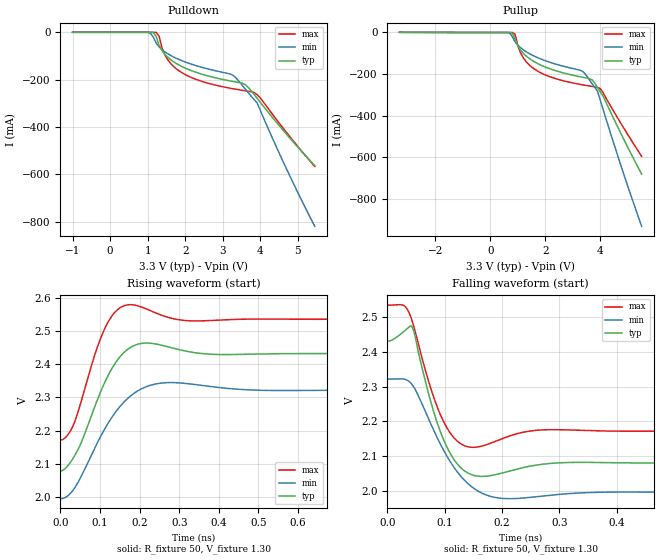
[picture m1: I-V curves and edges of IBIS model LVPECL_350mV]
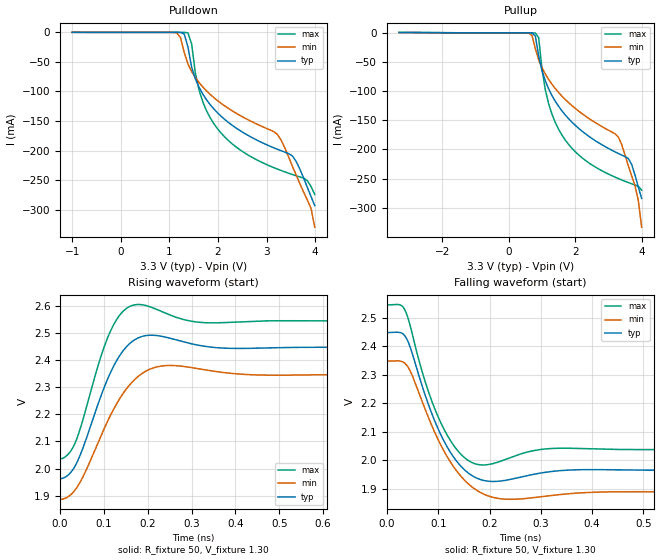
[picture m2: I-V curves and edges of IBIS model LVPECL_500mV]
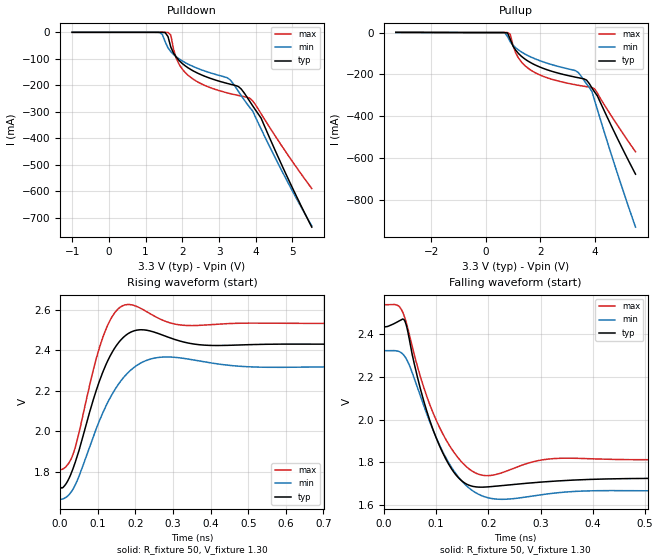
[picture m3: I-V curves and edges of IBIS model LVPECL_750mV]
|   This file is an IBIS representation of the   |
|   Integrated Device Technology Inc   |
|   8V49NS0312   |
|   FEMTOCLOCK NG CLOCK GENERATOR WITH 4 DIVIDERS   |
[IBIS Ver]   4.1
[File name]   8v49ns0312.ibs
[File Rev]   1.1
|Rev 1.1
|  Updated SDATA pin to I/O
|  Updated SCL Pin to SERIAL_IN
|Rev 1.0 Original, 13 Jun 2016
[Date]   01 Nov 2017
[Source]   Originated at Integrated Device Technology, Inc.
[Disclaimer]
IDT hereby grants the user of this IBIS model a non-exclusive,
nontransferable license to use this IBIS model under the following terms.
Before using this IBIS model, the user should read this license.
If the user does not accept these terms,  the IBIS model should be
returned to IDT within 30 days.
   The user is granted this license only to use the IBIS model and
is not granted rights to sell, load, rent, lease or license the IBIS
model in whole or in part, or in modified form to anyone other than
user. User may modify the IBIS model to suit its specific
applications but rights to derivative works and such modifications
shall belong to IDT.
   This IBIS model is provided on an "AS IS" basis and IDT makes
absolutely no warranty with respect to the information contained
herein. IDT DISCLAIMS AND CUSTOMER WAIVES ALL WARRANTIES, EXPRESS
OR IMPLIED, INCLUDING WARRANTIES OF MERCHANTABILITY OR FITNESS FOR
A PARTICULAR PURPOSE. The entire risk as to quality and performance
is with the Customer. ACCORDINGLY, IN NO EVENT SHALL THE COMPANY BE
LIABLE FOR ANY DAMAGES, WHETHER IN CONTRACT OR TORT,INCLUDING ANY
LOST PROFITS OR OTHER INCIDENTAL, CONSEQUENTIAL, EXEMPLARY, OR
PUNITIVE DAMAGES ARISING OUT OF THE USE OR APPLICATION OF THE IBIS
model provided in this package. Further, IDT reserves the right to
make changes without notice to any product herein to improve
reliability, function, or design. IDT does not convey any license
under patent rights or any other intellectual property rights,
including those of third parties.
   IDT is not obligated to provide maintenance or support
for the licensed IBIS model.
[Copyright] Copyright 2015 by Integrated Device Technology, Inc.
[Component]   8V49NS0312NLGI
[Manufacturer] Integrated Device Technology, Inc.
[Package]
|LD QFN 64
|lead + wire
|   Typ   Min   Max
R_pkg   0.15994   0.09324   0.20004
L_pkg   2.530359n   1.8988n   3.1063n
C_pkg   0.078001p   0.067589p   0.11523p
[Pin] signal_name model_name   R_pin   L_pin   C_pin
1  VCCOB   POWER   1.6449E-01   2.956n   0.08458p
2  QB0   LVDS_LVPECL_0312   1.9750E-01   2.7461n   0.088784p
3  nQB0   LVDS_LVPECL_0312   1.7981E-01   2.699n   0.082304p
4  QB1   LVDS_LVPECL_0312   1.7541E-01   2.4836n   0.082529p
5  nQB1   LVDS_LVPECL_0312   1.5766E-01   2.437n   0.075279p
6  QB2   LVDS_LVPECL_0312   1.4595E-01   2.3494n   0.071373p
7  nQB2   LVDS_LVPECL_0312   1.4009E-01   2.2382n   0.070004p
8  QB3   LVDS_LVPECL_0312   1.4152E-01   2.1201n   0.069711p
9  nQB3   LVDS_LVPECL_0312   1.4111E-01   2.1159n   0.069506p
10 VCCOB   POWER   1.3903E-01   2.2556n   0.069921p
11 ND[0]   RF_INESD_200_PUP   1.4414E-01   2.3769n   0.069368p
12 NC[1]   RF_INESD_200_PUP   1.4772E-01   2.3318n   0.070114p
13 VCCOD   POWER   1.5989E-01   2.3679n   0.077159p
14 QD1   RF_COUT_9F_7F_SE   1.6857E-01   2.5122n   0.077263p
15 QD0   LVDS_LVPECL_0312   1.6231E-01   2.543n   0.081562p
16 nQD0   LVDS_LVPECL_0312   1.3552E-01   2.8375n   0.077893p
17 NB[0]   RF_INESD_200_PUP   1.3290E-01   2.7501n   0.074621p
18 NB[1]   RF_INESD_200_PUP   1.8095E-01   2.7617n   0.08237p
19 NC[0]   RF_INESD_200_PUP   1.6926E-01   2.5289n   0.080624p
20 NC[1]   RF_INESD_200_PUP   1.6506E-01   2.3465n   0.075995p
21 VCCA_IN1   POWER   1.5450E-01   2.3031n   0.072045p
22 NA[1]   RF_INESD_200_PUP   1.4838E-01   2.1982n   0.072043p
23 CAPBIAS   NC   1.3877E-01   2.2149n   0.068646p
24 VCCA_IN2   POWER   1.3433E-01   2.1808n   0.068017p
25 CR   NC   1.4411E-01   2.1294n   0.070068p
26 CAPREG   NC   1.4387E-01   2.2043n   0.071183p
27 LFFR   NC   1.5194E-01   2.3838n   0.071178p
28 LFF   NC   1.5971E-01   2.3509n   0.075039p
29 VCCA   POWER   1.7026E-01   2.5352n   0.080161p
30 NC   NC   1.8017E-01   2.758n   0.086153p
31 VCC_CP   POWER   9.3242E-02   1.8988n   0.11523p
32 ICP   NC   1.3198E-01   2.7827n   0.071584p
33 VCCOC   POWER   1.6203E-01   3.0318n   0.081581p
34 nQC1   LVDS_LVPECL_0312   1.9612E-01   2.7713n   0.087674p
35 QC1   LVDS_LVPECL_0312   1.8463E-01   2.711n   0.082141p
36 nQC0   LVDS_LVPECL_0312   1.7410E-01   2.5236n   0.081436p
37 QC0   LVDS_LVPECL_0312   1.5857E-01   2.4566n   0.075124p
38 VCCOC   POWER   1.4575E-01   2.3561n   0.072098p
39 VCCOA   POWER   1.4055E-01   2.251n   0.070146p
40 nQA3   LVDS_LVPECL_0312   1.4352E-01   2.1244n   0.068826p
41 QA3   LVDS_LVPECL_0312   1.4468E-01   2.1039n   0.069621p
42 nQA2   LVDS_LVPECL_0312   1.3923E-01   2.2333n   0.067589p
43 QA2   LVDS_LVPECL_0312   1.4807E-01   2.2049n   0.069987p
44 nQA1   LVDS_LVPECL_0312   1.5598E-01   2.3003n   0.074857p
45 QA1   LVDS_LVPECL_0312   1.6074E-01   2.5324n   0.077114p
46 nQA0   LVDS_LVPECL_0312   1.7421E-01   2.6897n   0.082311p
47 QA0   LVDS_LVPECL_0312   2.0004E-01   2.7944n   0.09063p
48 VCCOA   POWER   1.6631E-01   3.0273n   0.085515p
49 REF_SEL   RF_INESD_200_PD   1.5017E-01   3.0793n   0.080972p
50 VCC_CK   POWER   1.7648E-01   2.7832n   0.08889p
51 nCLK   RF_INESD_200_PUP   1.9178E-01   2.7299n   0.087693p
52 CLK   RF_INESD_200_PD   1.7825E-01   2.7642n   0.082129p
53 FIN[1]   RF_INESD_200_PUP   1.6637E-01   2.7168n   0.080022p
54 FIN[0]   RF_INESD_200_PUP   1.6226E-01   2.6712n   0.0769p
55 CAPXTAL   NC   1.5685E-01   2.6157n   0.07263p
56 OSCO   NC   1.6928E-01   2.4353n   0.077211p
57 OSCI   NC   1.6908E-01   2.4716n   0.079042p
58 VCCA_XT   POWER   1.6376E-01   2.5979n   0.078197p
59 NA[0]   RF_INESD_200_PUP   1.7407E-01   2.5694n   0.081073p
60 RES   NC   1.7923E-01   2.6937n   0.079745p
61 SDATA   SERIAL_IO   1.7655E-01   2.8937n   0.079001p
62 SCLK   SERIAL_IN   1.8689E-01   2.9915n   0.086026p
63 VCC_SP   POWER   1.7813E-01   3.1063n   0.089577p
64 LOCK   RF_COUT_12F_IO   1.6199E-01   3.0138n   0.083996p
[Diff Pin]   inv_pin vdiff   tdelay_typ   tdelay_min   tdelay_max
| Inputs
52   51   0.2   NA   NA   NA
|Outputs
2   3   NA   0   0   0
4   5   NA   0   0   0
6   7   NA   0   0   0
8   9   NA   0   0   0
15   16   NA   0   0   0
47   46   NA   0   0   0
45   44   NA   0   0   0
43   42   NA   0   0   0
41   40   NA   0   0   0
37   36   NA   0   0   0
35   34   NA   0   0   0
[Model Selector] LVDS_LVPECL_0312
LVDS_350mV   350mV LVDS Model
LVDS_500mV   500mV LVDS Model
LVDS_750mV   750mV LVDS Model
LVPECL_350mV   350mV LVPECL Model
LVPECL_500mV   500mV LVPECL Model
LVPECL_750mV   750mV LVPECL Model
| Models and submodels in the file (12): LVPECL_350mV (Output_ECL), LVPECL_500mV (Output_ECL), LVPECL_750mV (Output_ECL), LVDS_350mV (Output), LVDS_500mV (Output), LVDS_750mV (Output), RF_INESD_200_PUP (Input), RF_COUT_9F_7F_SE (Output), RF_INESD_200_PD (Input), RF_COUT_12F_IO (Output), SERIAL_IO (I/O_open_drain), SERIAL_IN (Input)
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[Model]   LVPECL_350mV
Model_type   Output_ECL
Polarity   Non-Inverting
|   typ   min   max
C_comp   2pF   1.5pF   2.5pF
Vmeas= 2.244V
Rref = 50
Cref = 0
Vref = 1.3V
|   typ   min   max
[Voltage range]   3.3V   3.135V   3.465V
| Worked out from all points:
|   rising waveform, R_fixture 50, V_fixture 1.30: 20-80 % time 71.2ps typ, 87.9ps min, 55.4ps max; typ from 2.08 V to 2.43 V
|   falling waveform, R_fixture 50, V_fixture 1.30: 20-80 % time 37.7ps typ, 60.2ps min, 38.3ps max; typ from 2.43 V to 2.08 V
[Pulldown]
|Voltage   I (typ)   I (min)   I (max)
-1V       46.99uA    55.49uA    39.05uA
996mV     -2.417uA   -292.3uA   -6.854nA
1.226V    -17.75mA   -46.05mA   -610.7uA
1.303V    -54.71mA   -61.43mA   -16.42mA
1.38V     -76.94mA   -72.91mA   -65.09mA
1.533V    -105.1mA   -90.45mA   -115.9mA
1.84V     -139mA     -115.4mA   -163.4mA
3.299V    -208.7mA   -185mA     -239.4mA
3.606V    -222.3mA   -241.7mA   -247.6mA
3.913V    -278.8mA   -298.2mA   -263.6mA
4.681V    -427.9mA   -572.1mA   -420.1mA
5.448V    -563mA     -819.9mA   -567.2mA
[Pullup]
|Voltage   I (typ)   I (min)   I (max)
-3.3V     781.4uA    613.4uA    1.002mA
600mV     -980.9nA   -86.79uA   -5.239nA
800mV     -2.307mA   -19.53mA   -84.09uA
900mV     -32.62mA   -44.9mA    -8.184mA
1V        -64.66mA   -60.7mA    -61.81mA
1.2V      -100.1mA   -83.16mA   -121.4mA
1.6V      -140.4mA   -113.6mA   -175.2mA
3.4V      -216.2mA   -191.5mA   -252.3mA
3.7V      -227.4mA   -246mA     -258.9mA
3.9V      -265.1mA   -282.8mA   -263.2mA
4.1V      -304.9mA   -369.6mA   -289.4mA
5.5V      -679.8mA   -930.4mA   -594.4mA
[Ramp]
|   typ   min   max
dV/dt_r   0.23/0.08n   0.209/0.098n   0.244/0.064n
dV/dt_f   0.26/0.047n   0.207/0.066n   0.247/0.046n
R_load =   50.0000
[Rising Waveform]
R_fixture = 50
V_fixture = 1.30   | VCC_typ - 2V
V_fixture_max = 1.465   | VCC_max - 2V
V_fixture_min = 1.135   | VCC_min - 2V
C_fixture = 0.0p
| Time   typ   min   max
0s        2.08V      1.995V     2.172V
34.03ps   2.121V     2.024V     2.221V
88.09ps   2.277V     2.151V     2.433V
114.1ps   2.351V     2.21V      2.512V
140.1ps   2.406V     2.257V     2.559V
168.2ps   2.443V     2.295V     2.578V
212.2ps   2.463V     2.33V      2.568V
276.3ps   2.451V     2.344V     2.539V
406.4ps   2.429V     2.329V     2.533V
2ns       2.431V     2.322V     2.535V
[Falling Waveform]
R_fixture = 50
V_fixture = 1.30   | VCC_typ - 2V
V_fixture_max = 1.465   | VCC_max - 2V
V_fixture_min = 1.135   | VCC_min - 2V
C_fixture = 0.0p
| Time   typ   min   max
0s        2.432V     2.322V     2.535V
30.03ps   2.461V     2.322V     2.533V
44.04ps   2.47V      2.304V     2.486V
72.07ps   2.279V     2.207V     2.315V
94.09ps   2.163V     2.129V     2.214V
118.1ps   2.086V     2.063V     2.149V
144.1ps   2.048V     2.015V     2.126V
194.2ps   2.049V     1.979V     2.146V
280.3ps   2.078V     1.986V     2.176V
2ns       2.08V      1.996V     2.172V
[Model]   LVPECL_500mV
Model_type   Output_ECL
Polarity   Non-Inverting
|   typ   min   max
C_comp   2pF   1.5pF   2.5pF
Vmeas= 2.203V
Rref = 50
Cref = 0
Vref = 1.3V
|   typ   min   max
[Voltage range]   3.3V   3.135V   3.465V
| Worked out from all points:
|   rising waveform, R_fixture 50, V_fixture 1.30: 20-80 % time 65.5ps typ, 80ps min, 55.1ps max; typ from 1.96 V to 2.45 V
|   falling waveform, R_fixture 50, V_fixture 1.30: 20-80 % time 59.8ps typ, 70.6ps min, 53.8ps max; typ from 2.45 V to 1.96 V
[Pulldown]
|Voltage   I (typ)   I (min)   I (max)
|Note, modeling breaks down at 250mA and above.  This is well beyond the functional   |
|operating range of the device.  Should this scenario occur, catastrophic failure and   |
|possible damage to the device and/or board is of higher concern than the I-V curve   |
|behavior.  The IBIS checker will flag currents in excess of 10A with warnings.  Lines   |
|with currents in excess of 0.35 A have been commented out.  The points still remain|
|available to the user if the user desires to use them.   |
|Note, modeling breaks down at 250mA and above.  This is well beyond the functional   |
|operating range of the device.  Should this scenario occur, catastrophic failure and   |
|possible damage to the device and/or board is of higher concern than the I-V curve   |
|behavior.  The IBIS checker will flag currents in excess of 10A with warnings.  Lines   |
|with currents in excess of 0.35 A have been commented out.  The points still remain|
|available to the user if the user desires to use them.   |
-1V       49.32uA    57.22uA    39.05uA
1.149V    -6.032uA   -1.009mA   -8.922nA
1.303V    -2.562mA   -33.63mA   -17.79uA
1.38V     -24.61mA   -53.43mA   -796.1uA
1.457V    -59.03mA   -66.37mA   -19.68mA
1.533V    -78.83mA   -76.55mA   -69.1mA
1.687V    -104.7mA   -92.49mA   -117.8mA
2.071V    -142.6mA   -120.6mA   -171.2mA
3.222V    -198mA     -172.8mA   -231.5mA
3.606V    -218.3mA   -241.5mA   -242.7mA
3.913V    -277.9mA   -297.8mA   -260.9mA
3.99V     -293.3mA   -329.8mA   -274.5mA
|| 4.06667e+00   -3.08432e-01   -3.67426e-01   -2.90478e-01
|| 4.14343e+00   -3.23924e-01   -4.05071e-01   -3.07173e-01
|| 4.22020e+00   -3.53714e-01   -4.42647e-01   -3.23828e-01
|| 4.29697e+00   -3.97748e-01   -4.80134e-01   -3.40232e-01
|| 4.37374e+00   -4.42041e-01   -5.17517e-01   -3.56685e-01
|| 4.45051e+00   -4.86426e-01   -5.54778e-01   -3.88442e-01
|| 4.52727e+00   -5.30804e-01   -5.91886e-01   -4.43339e-01
|| 4.60404e+00   -5.75132e-01   -5.91886e-01   -4.97475e-01
|| 4.68081e+00   -6.19384e-01   -5.91886e-01   -5.50215e-01
|| 4.75758e+00   -6.63538e-01   -5.91886e-01   -6.03199e-01
|| 4.83434e+00   -7.07558e-01   -5.91886e-01   -6.56255e-01
|| 4.91111e+00   -7.51390e-01   -5.91886e-01   -7.09286e-01
|| 4.98788e+00   -7.94950e-01   -5.91886e-01   -7.62250e-01
|| 5.06465e+00   -8.38293e-01   -5.91886e-01   -8.15110e-01
|| 5.14141e+00   -8.38293e-01   -5.91886e-01   -8.67827e-01
|| 5.21818e+00   -8.38293e-01   -5.91886e-01   -9.20344e-01
|| 5.29495e+00   -8.38293e-01   -5.91886e-01   -9.72672e-01
|| 5.37172e+00   -8.38293e-01   -5.91886e-01   -1.02500e+00
|| 5.44848e+00   -8.38293e-01   -5.91886e-01   -1.07696e+00
[Pullup]
|Voltage   I (typ)   I (min)   I (max)
|Note, modeling breaks down at 250mA and above.  This is well beyond the functional   |
|operating range of the device.  Should this scenario occur, catastrophic failure and   |
|possible damage to the device and/or board is of higher concern than the I-V curve   |
|behavior.  The IBIS checker will flag currents in excess of 10A with warnings.  Lines   |
|with currents in excess of 0.35 A have been commented out.  The points still remain|
|available to the user if the user desires to use them.   |
-3.3V     746.6uA    586.4uA    1.002mA
700mV     -165.7uA   -4.504mA   -647nA
800mV     -5.314mA   -26.92mA   -83.98uA
900mV     -39.18mA   -46.19mA   -8.176mA
1V        -64.77mA   -59.66mA   -61.8mA
1.2V      -95.95mA   -79.87mA   -121.4mA
1.7V      -140.7mA   -114.2mA   -183.7mA
3.3V      -206.9mA   -178.8mA   -249.9mA
3.6V      -215.6mA   -228mA     -256.8mA
3.8V      -243.9mA   -262.2mA   -261mA
3.9V      -264.5mA   -287.2mA   -263.2mA
4V        -283.9mA   -333.3mA   -269.8mA
| 4.10000e+00   -3.02415e-01   -3.78849e-01   -2.89415e-01
| 4.20000e+00   -3.40057e-01   -4.23937e-01   -3.13568e-01
| 4.30000e+00   -3.94775e-01   -4.68570e-01   -3.35833e-01
| 4.40000e+00   -4.49108e-01   -4.68570e-01   -3.56546e-01
| 4.50000e+00   -5.03021e-01   -4.68570e-01   -4.17084e-01
| 4.60000e+00   -5.56418e-01   -4.68570e-01   -4.85623e-01
| 4.70000e+00   -6.09244e-01   -4.68570e-01   -5.54012e-01
| 4.80000e+00   -6.61642e-01   -4.68570e-01   -6.22199e-01
| 4.90000e+00   -7.13735e-01   -4.68570e-01   -6.90136e-01
| 5.00000e+00   -7.13735e-01   -4.68570e-01   -7.57722e-01
| 5.10000e+00   -7.13735e-01   -4.68570e-01   -8.24630e-01
| 5.20000e+00   -7.13735e-01   -4.68570e-01   -8.90368e-01
| 5.30000e+00   -7.13735e-01   -4.68570e-01   -9.55440e-01
| 5.40000e+00   -7.13735e-01   -4.68570e-01   -1.02066e+00
| 5.50000e+00   -7.13735e-01   -4.68570e-01   -1.08596e+00
[Ramp]
|   typ   min   max
dV/dt_r   0.316/0.074n   0.295/0.088n   0.34/0.064n
dV/dt_f   0.314/0.068n   0.291/0.077n   0.338/0.064n
R_load =   50.0000
[Rising Waveform]
R_fixture = 50
V_fixture = 1.30   | VCC_typ - 2V
V_fixture_max = 1.465   | VCC_max - 2V
V_fixture_min = 1.135   | VCC_min - 2V
C_fixture = 0.0p
| Time   typ   min   max
0s        1.963V     1.887V     2.036V
20.02ps   1.979V     1.898V     2.056V
36.04ps   2.015V     1.925V     2.101V
92.09ps   2.263V     2.117V     2.408V
118.1ps   2.365V     2.207V     2.518V
142.1ps   2.431V     2.273V     2.577V
170.2ps   2.474V     2.328V     2.603V
234.2ps   2.486V     2.378V     2.577V
340.3ps   2.448V     2.361V     2.537V
2ns       2.446V     2.346V     2.544V
[Falling Waveform]
R_fixture = 50
V_fixture = 1.30   | VCC_typ - 2V
V_fixture_max = 1.465   | VCC_max - 2V
V_fixture_min = 1.135   | VCC_min - 2V
C_fixture = 0.0p
| Time   typ   min   max
0s        2.448V     2.348V     2.545V
26.03ps   2.448V     2.348V     2.545V
36.04ps   2.433V     2.338V     2.523V
80.08ps   2.199V     2.153V     2.244V
118.1ps   2.044V     2.01V      2.086V
148.1ps   1.971V     1.935V     2.013V
180.2ps   1.933V     1.888V     1.984V
234.2ps   1.93V      1.863V     2.005V
336.3ps   1.963V     1.879V     2.042V
2ns       1.964V     1.888V     2.037V
[Model]   LVPECL_750mV
Model_type   Output_ECL
Polarity   Non-Inverting
|   typ   min   max
C_comp   2pF   1.5pF   2.5pF
Vmeas= 2.084V
Rref = 50
Cref = 0
Vref = 1.3V
|   typ   min   max
[Voltage range]   3.3V   3.135V   3.465V
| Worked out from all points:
|   rising waveform, R_fixture 50, V_fixture 1.30: 20-80 % time 69.3ps typ, 86ps min, 55.4ps max; typ from 1.73 V to 2.43 V
|   falling waveform, R_fixture 50, V_fixture 1.30: 20-80 % time 52.9ps typ, 66ps min, 58.3ps max; typ from 2.43 V to 1.73 V
[Pulldown]
|Voltage   I (typ)   I (min)   I (max)
-1V       46.99uA    52.79uA    34.37uA
1.38V     -1.938uA   -734uA     -1.297nA
1.457V    -46.63uA   -8.101mA   -69.37nA
1.61V     -15.95mA   -58.81mA   -244.4uA
1.687V    -55.72mA   -73.05mA   -10.72mA
1.84V     -94.89mA   -92.95mA   -100.1mA
2.147V    -133.2mA   -119.4mA   -161mA
3.222V    -193mA     -171.6mA   -228.6mA
3.529V    -204.9mA   -223.5mA   -238.6mA
3.913V    -276.9mA   -296.7mA   -258.7mA
4.143V    -323.6mA   -364.6mA   -307mA
5.525V    -736mA     -731.5mA   -590.1mA
[Pullup]
|Voltage   I (typ)   I (min)   I (max)
-3.3V     781.4uA    613.4uA    1.002mA
600mV     -965.4nA   -83.72uA   -5.214nA
800mV     -2.274mA   -19.17mA   -83.69uA
900mV     -32.44mA   -44.7mA    -8.155mA
1V        -64.57mA   -60.56mA   -61.77mA
1.2V      -100mA     -83.07mA   -121.4mA
1.6V      -140.4mA   -113.6mA   -175.2mA
3.4V      -216.2mA   -191.4mA   -252.3mA
3.7V      -227.4mA   -245.4mA   -258.9mA
3.9V      -265.1mA   -282.1mA   -263.2mA
4.1V      -303.3mA   -369mA     -289.4mA
5.5V      -677.6mA   -930.8mA   -570.3mA
[Ramp]
|   typ   min   max
dV/dt_r   0.468/0.08n   0.421/0.097n   0.489/0.065n
dV/dt_f   0.47/0.059n   0.416/0.072n   0.478/0.07n
R_load =   50.0000
[Rising Waveform]
R_fixture = 50
V_fixture = 1.30   | VCC_typ - 2V
V_fixture_max = 1.465   | VCC_max - 2V
V_fixture_min = 1.135   | VCC_min - 2V
C_fixture = 0.0p
| Time   typ   min   max
0s        1.725V     1.665V     1.811V
36.04ps   1.826V     1.721V     1.897V
92.09ps   2.181V     1.995V     2.332V
120.1ps   2.323V     2.119V     2.497V
146.1ps   2.415V     2.209V     2.588V
174.2ps   2.474V     2.278V     2.625V
244.2ps   2.493V     2.359V     2.576V
340.3ps   2.436V     2.357V     2.523V
548.5ps   2.43V      2.317V     2.534V
2ns       2.431V     2.319V     2.533V
[Falling Waveform]
R_fixture = 50
V_fixture = 1.30   | VCC_typ - 2V
V_fixture_max = 1.465   | VCC_max - 2V
V_fixture_min = 1.135   | VCC_min - 2V
C_fixture = 0.0p
| Time   typ   min   max
0s        2.432V     2.321V     2.535V
26.03ps   2.456V     2.319V     2.533V
40.04ps   2.46V      2.294V     2.474V
76.08ps   2.088V     2.066V     2.151V
112.1ps   1.847V     1.852V     1.936V
148.1ps   1.716V     1.716V     1.804V
190.2ps   1.685V     1.642V     1.74V
234.2ps   1.694V     1.628V     1.759V
342.3ps   1.715V     1.661V     1.82V
2ns       1.726V     1.667V     1.813V
